(* Logix 5000 AddOnInstructionDefinition export; software revision 16.00 *)

ADD_ON_INSTRUCTION AMCI_ANG1E_Disable_Driver   (* revision 1.0, vendor AMCI *)
VAR_IN_OUT
   AMCI_ANG1E_output_data : INT[10]; {required}
END_VAR
VAR
   command_data_block : INT[10];
        [0]   // Command Bits MSW
        [1]   // Command Bits LSW
        [2]   // Upper Target Position
        [3]   // Lower Target Position
        [4]   // Upper Programmed Speed
        [5]   // Lower Programmed Speed
END_VAR

ROUTINE Logic   (* ladder *)
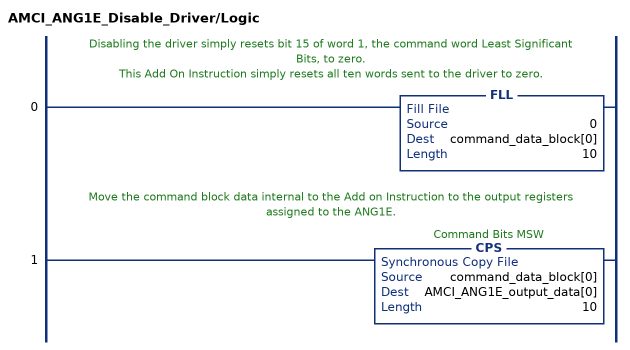
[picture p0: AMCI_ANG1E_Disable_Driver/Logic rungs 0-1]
   // Disabling the driver simply resets bit 15 of word 1, the command word Least Significant Bits, to zero.
   // This Add On Instruction simply resets all ten words sent to the driver to zero.
   0: FLL(0,command_data_block[0],10);
   // Move the command block data internal to the Add on Instruction to the output registers assigned to the ANG1E.
   1: CPS(command_data_block[0],AMCI_ANG1E_output_data[0],10);
END_ROUTINE
END_ADD_ON_INSTRUCTION
